(* Logix 5000 AddOnInstructionDefinition export Banner_IOL_Parameter_v6; software revision 33.00 *)

TYPE Banner_IOL_Device_Index_v6 :
STRUCT
   Index : Banner_IOL_Device_SubIndex_v6[41];
END_STRUCT
END_TYPE

TYPE Banner_IOL_Device_SubIndex_v6 :
STRUCT
   Sub : DINT[34];
END_STRUCT
END_TYPE

TYPE Banner_IOL_Device_v6 :
STRUCT
   Initial_Global_Read : BOOL;
   Command : SINT;
   Data : Banner_IOL_Device_Index_v6;
   Reset : BOOL;
END_STRUCT
END_TYPE

TYPE Banner_IOL_Port_v6 :   // UDT that has all of the data items necessary to communicate with a specific Port on a IO-Link Master
STRUCT
   Port_Controlled : INT;   // Each bit represents a port on an IO-Link Master. Set to 1 to tell AOI to control that port.
   Port_Activate : INT;   // Each bit represents a port on an IO-Link Master. When ON that port will process any commands in queue.
   Port_Read : INT;   // Each bit represents a port on an IO-Link Master. Used to determine when device AOI has requested a Read command.
   Port_Write : INT;   // Each bit represents a port on an IO-Link Master. Used to determine when device AOI has requested a Write command.
   Port_RW_Complete : INT;   // Each bit represents a port on an IO-Link Master. Tells device AOI that Read or Write request has been completed.
   Port_Device_Read : INT;
   Data_Transfer : SINT[250];   // Array to transfer data from IO-Master to device AOIs.
END_STRUCT
END_TYPE

TYPE Banner_IOL_Rules_Array_v6 :
STRUCT
   Length : DINT;
   Settings : Banner_IOL_Rules_SettingsArray_v6[41];
END_STRUCT
END_TYPE

TYPE Banner_IOL_Rules_SettingsArray_v6 :
STRUCT
   Index : DINT;
   Sub_Index : DINT;
   Num_Op : INT;   // Number of Operations to read/write Index.
   Total_Bytes : INT;
   RW : SINT;   // 0 = Read Only, 1 = Write Only, 2 = Read or Write
   Rules : Banner_IOL_Rules_v6[34];   // Sub Index Position in IODD.
END_STRUCT
END_TYPE

TYPE Banner_IOL_Rules_v6 :
STRUCT
   Byte_Pos : SINT;   // Byte Position to read from or write data to.
   Multi : SINT;   // Determines if a multiple byte length index is being accessed. Use 2 for 2 bytes length, 3 for 3 byte length, etc..
   BitControl : BOOL;   // 0=Standard byte control, 1=Bitwise packaging
   BitPos : SINT;   // Bit start position for operation
   BitValue : SINT;
   Sub_Index : SINT;
   Signed : SINT;   // 0=Unsigned, 1=Signed
END_STRUCT
END_TYPE

ADD_ON_INSTRUCTION Banner_IOL_Parameter_v6   (* revision 6.0 *)
// AOI that reads and writes to an IO-Link devices parameter data.
VAR_IN_OUT
   Device : Banner_IOL_Device_v6; {required}
   Rules : Banner_IOL_Rules_Array_v6; {required}
   Port_Data : Banner_IOL_Port_v6; {required}
END_VAR
VAR_INPUT
   Port : DINT; {required}
END_VAR
VAR_OUTPUT
   Done : BOOL; {access Read Only, visible}
   Busy : BOOL; {access Read Only, visible}
END_VAR
VAR
   Control : DINT; {access None}
   Inprocess_Index : INT; {access None}
   Index_Write_Inprocess : INT; {access None}
   Index_Write_Control : INT; {access None}
   Global_Read_Command : INT; {access None}
   Command_Being_Processed : BOOL; {access None}
   r_dex2 : INT; {access None}
   r_dex1 : INT; {access None}
   g_index : INT; {access None}
   r_dex3 : INT; {access None}
   r_dex4 : INT; {access None}
   r_dex5 : INT; {access None}
   Wr_Upper : INT; {access None}
   w_dex5 : INT; {access None}
   w_dex4 : INT; {access None}
   w_dex3 : INT; {access None}
   w_dex2 : INT; {access None}
   w_dex1 : INT; {access None}
   m3 : INT; {access None}
   m2 : INT; {access None}
   m1 : INT; {access None}
   b_dex : INT; {access None}
   GlobalCon : DINT; {access None}
   Signed : INT; {access None}
   Temp_Int : INT; {access None}
   Temp_Write : DINT; {access None}
   Temp_Read : DINT; {access None}
   Temp : DINT[10]; {access None}
END_VAR

ROUTINE Logic   (* ladder *)
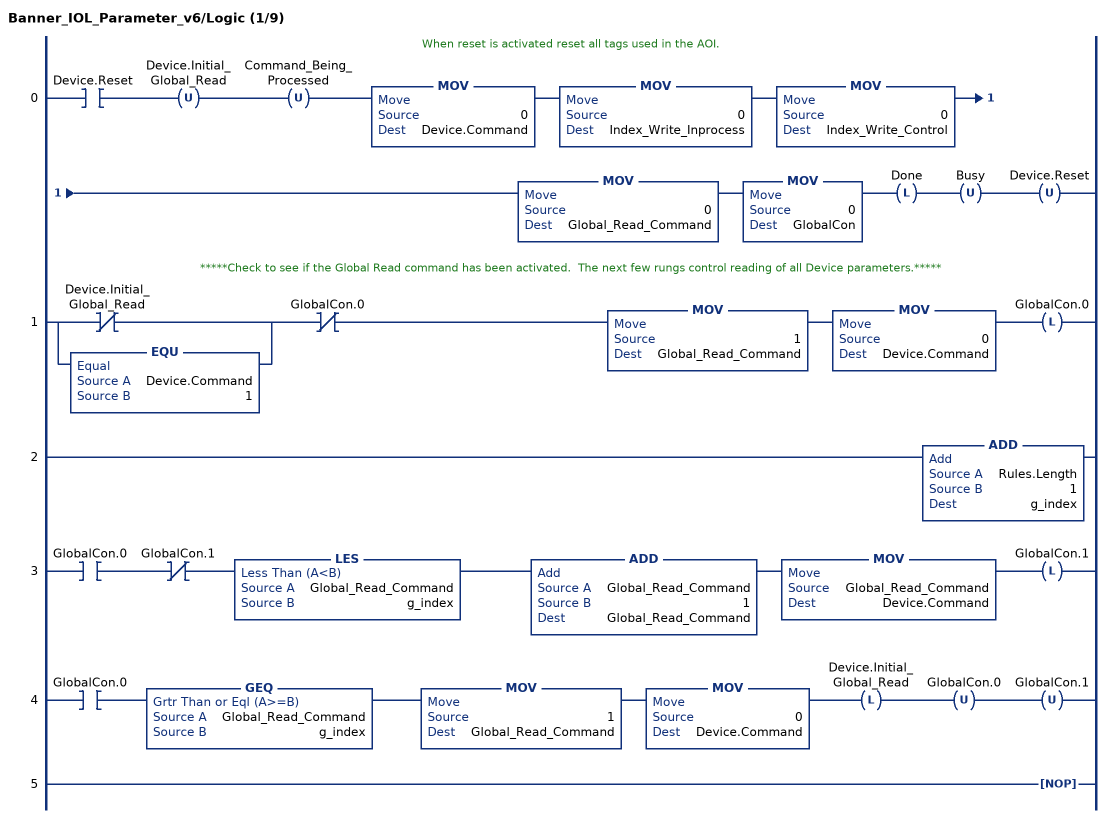
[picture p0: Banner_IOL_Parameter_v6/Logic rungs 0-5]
   // When reset is activated reset all tags used in the AOI.
   0: XIC(Device.Reset)OTU(Device.Initial_Global_Read)OTU(Command_Being_Processed)MOV(0,Device.Command)MOV(0,Index_Write_Inprocess)MOV(0,Index_Write_Control)MOV(0,Global_Read_Command)MOV(0,GlobalCon)OTL(Done)OTU(Busy)OTU(Device.Reset);
   // *****Check to see if the Global Read command has been activated.  The next few rungs control reading of all Device parameters.*****
   1: [XIO(Device.Initial_Global_Read) ,EQU(Device.Command,1) ]XIO(GlobalCon.0)MOV(1,Global_Read_Command)MOV(0,Device.Command)OTL(GlobalCon.0);
   2: ADD(Rules.Length,1,g_index);
   3: XIC(GlobalCon.0)XIO(GlobalCon.1)LES(Global_Read_Command,g_index)ADD(Global_Read_Command,1,Global_Read_Command)MOV(Global_Read_Command,Device.Command)OTL(GlobalCon.1);
   4: XIC(GlobalCon.0)GEQ(Global_Read_Command,g_index)MOV(1,Global_Read_Command)MOV(0,Device.Command)OTL(Device.Initial_Global_Read)OTU(GlobalCon.0)OTU(GlobalCon.1);
   5: NOP();
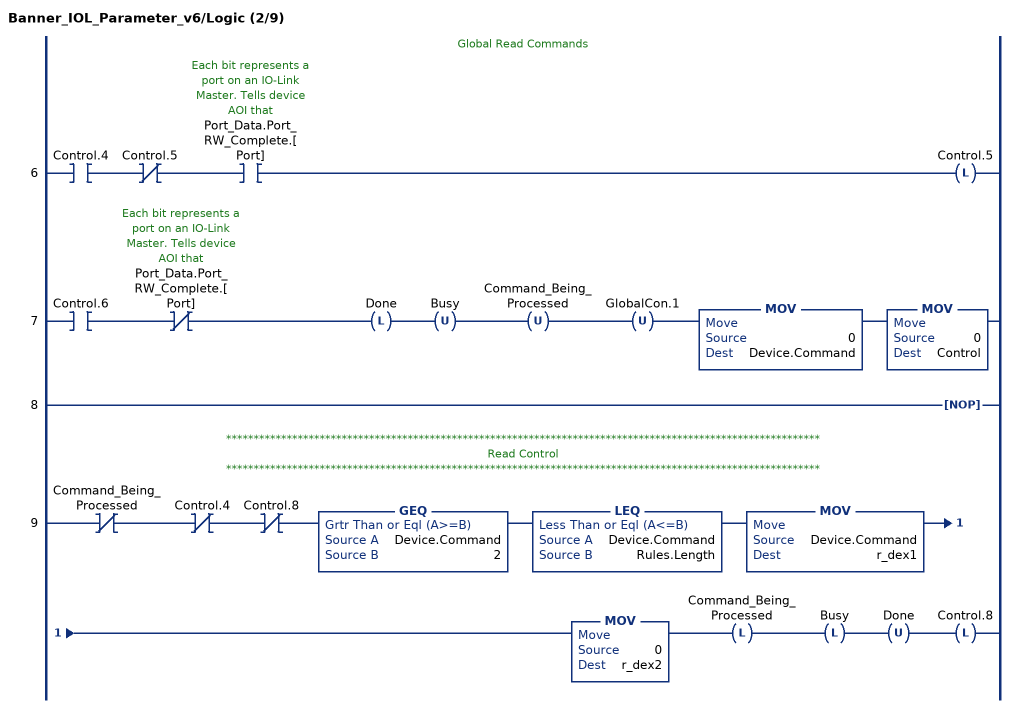
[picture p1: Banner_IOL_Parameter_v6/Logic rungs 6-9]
   // Global Read Commands
   6: XIC(Control.4)XIO(Control.5)XIC(Port_Data.Port_RW_Complete.[Port])OTL(Control.5);
   7: XIC(Control.6)XIO(Port_Data.Port_RW_Complete.[Port])OTL(Done)OTU(Busy)OTU(Command_Being_Processed)OTU(GlobalCon.1)MOV(0,Device.Command)MOV(0,Control);
   8: NOP();
   // ************************************************************************************************************
   // Read Control
   // ************************************************************************************************************
   9: XIO(Command_Being_Processed)XIO(Control.4)XIO(Control.8)GEQ(Device.Command,2)LEQ(Device.Command,Rules.Length)MOV(Device.Command,r_dex1)MOV(0,r_dex2)OTL(Command_Being_Processed)OTL(Busy)OTU(Done)OTL(Control.8);
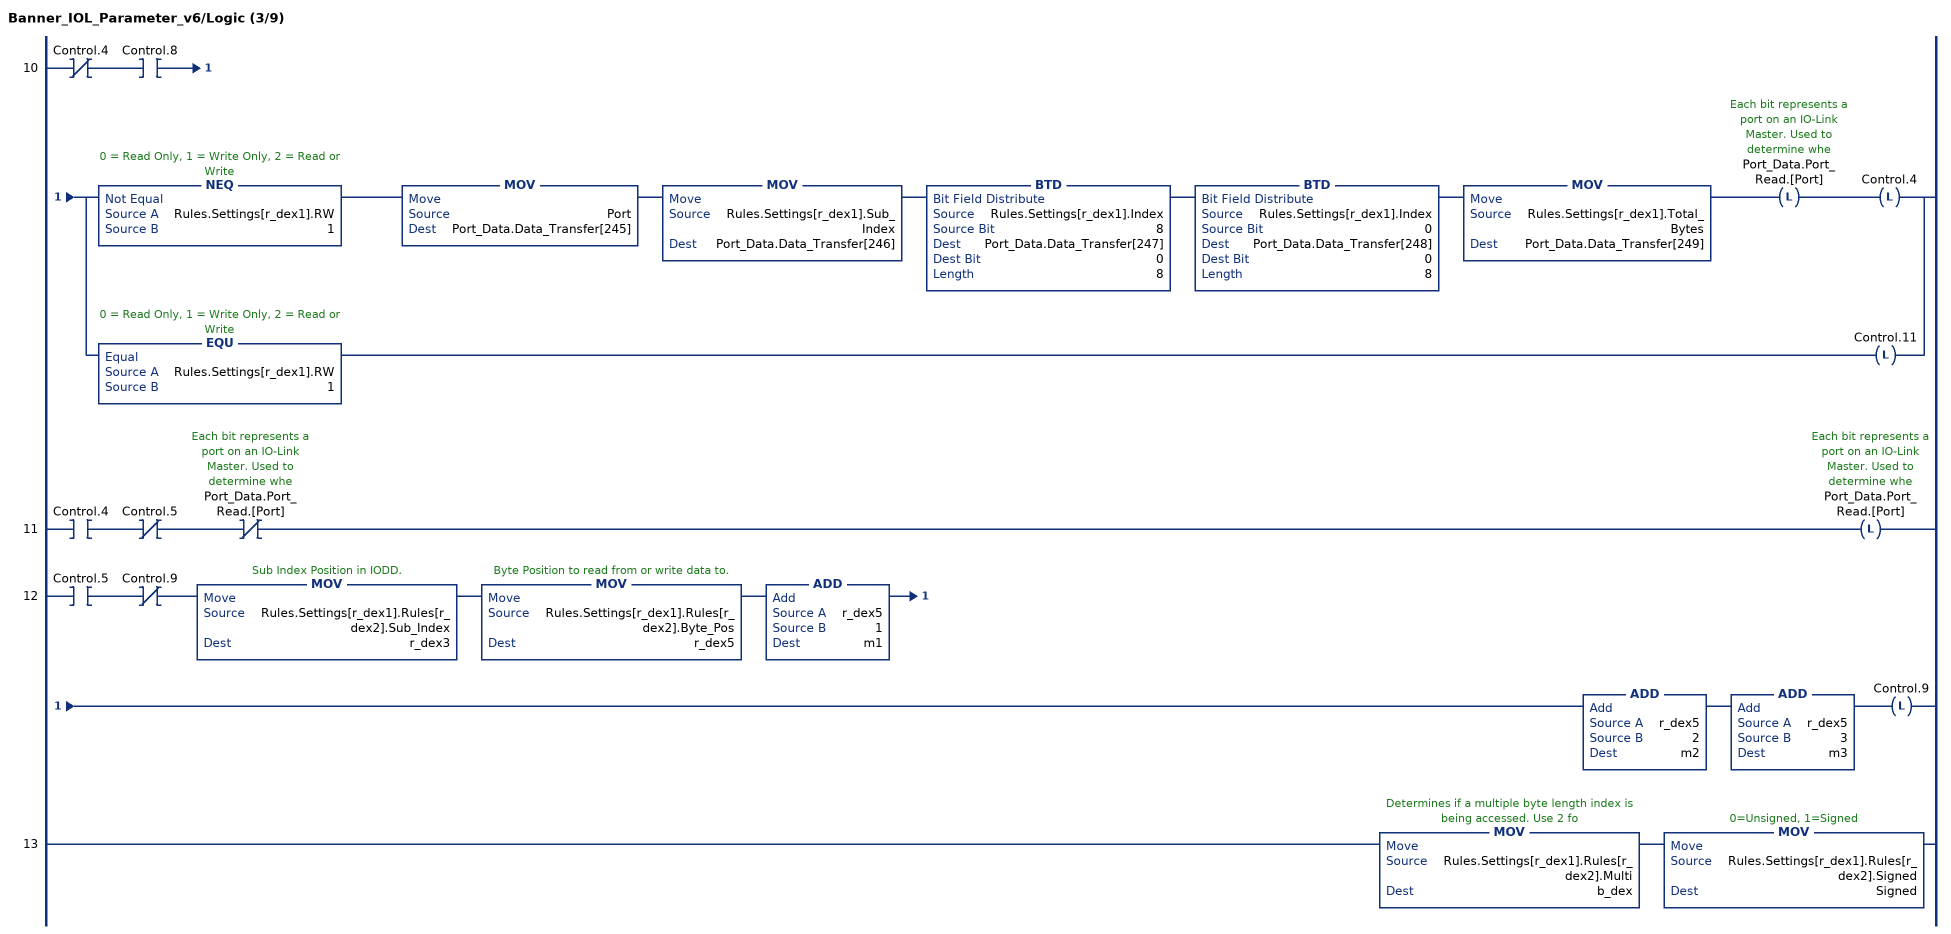
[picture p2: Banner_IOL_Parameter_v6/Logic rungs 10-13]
   10: XIO(Control.4)XIC(Control.8)[NEQ(Rules.Settings[r_dex1].RW,1) MOV(Port,Port_Data.Data_Transfer[245]) MOV(Rules.Settings[r_dex1].Sub_Index,Port_Data.Data_Transfer[246]) BTD(Rules.Settings[r_dex1].Index,8,Port_Data.Data_Transfer[247],0,8) BTD(Rules.Settings[r_dex1].Index,0,Port_Data.Data_Transfer[248],0,8) MOV(Rules.Settings[r_dex1].Total_Bytes,Port_Data.Data_Transfer[249]) OTL(Port_Data.Port_Read.[Port]) OTL(Control.4) ,EQU(Rules.Settings[r_dex1].RW,1) OTL(Control.11) ];
   11: XIC(Control.4)XIO(Control.5)XIO(Port_Data.Port_Read.[Port])OTL(Port_Data.Port_Read.[Port]);
   12: XIC(Control.5)XIO(Control.9)MOV(Rules.Settings[r_dex1].Rules[r_dex2].Sub_Index,r_dex3)MOV(Rules.Settings[r_dex1].Rules[r_dex2].Byte_Pos,r_dex5)ADD(r_dex5,1,m1)ADD(r_dex5,2,m2)ADD(r_dex5,3,m3)OTL(Control.9);
   13: MOV(Rules.Settings[r_dex1].Rules[r_dex2].Multi,b_dex)MOV(Rules.Settings[r_dex1].Rules[r_dex2].Signed,Signed);
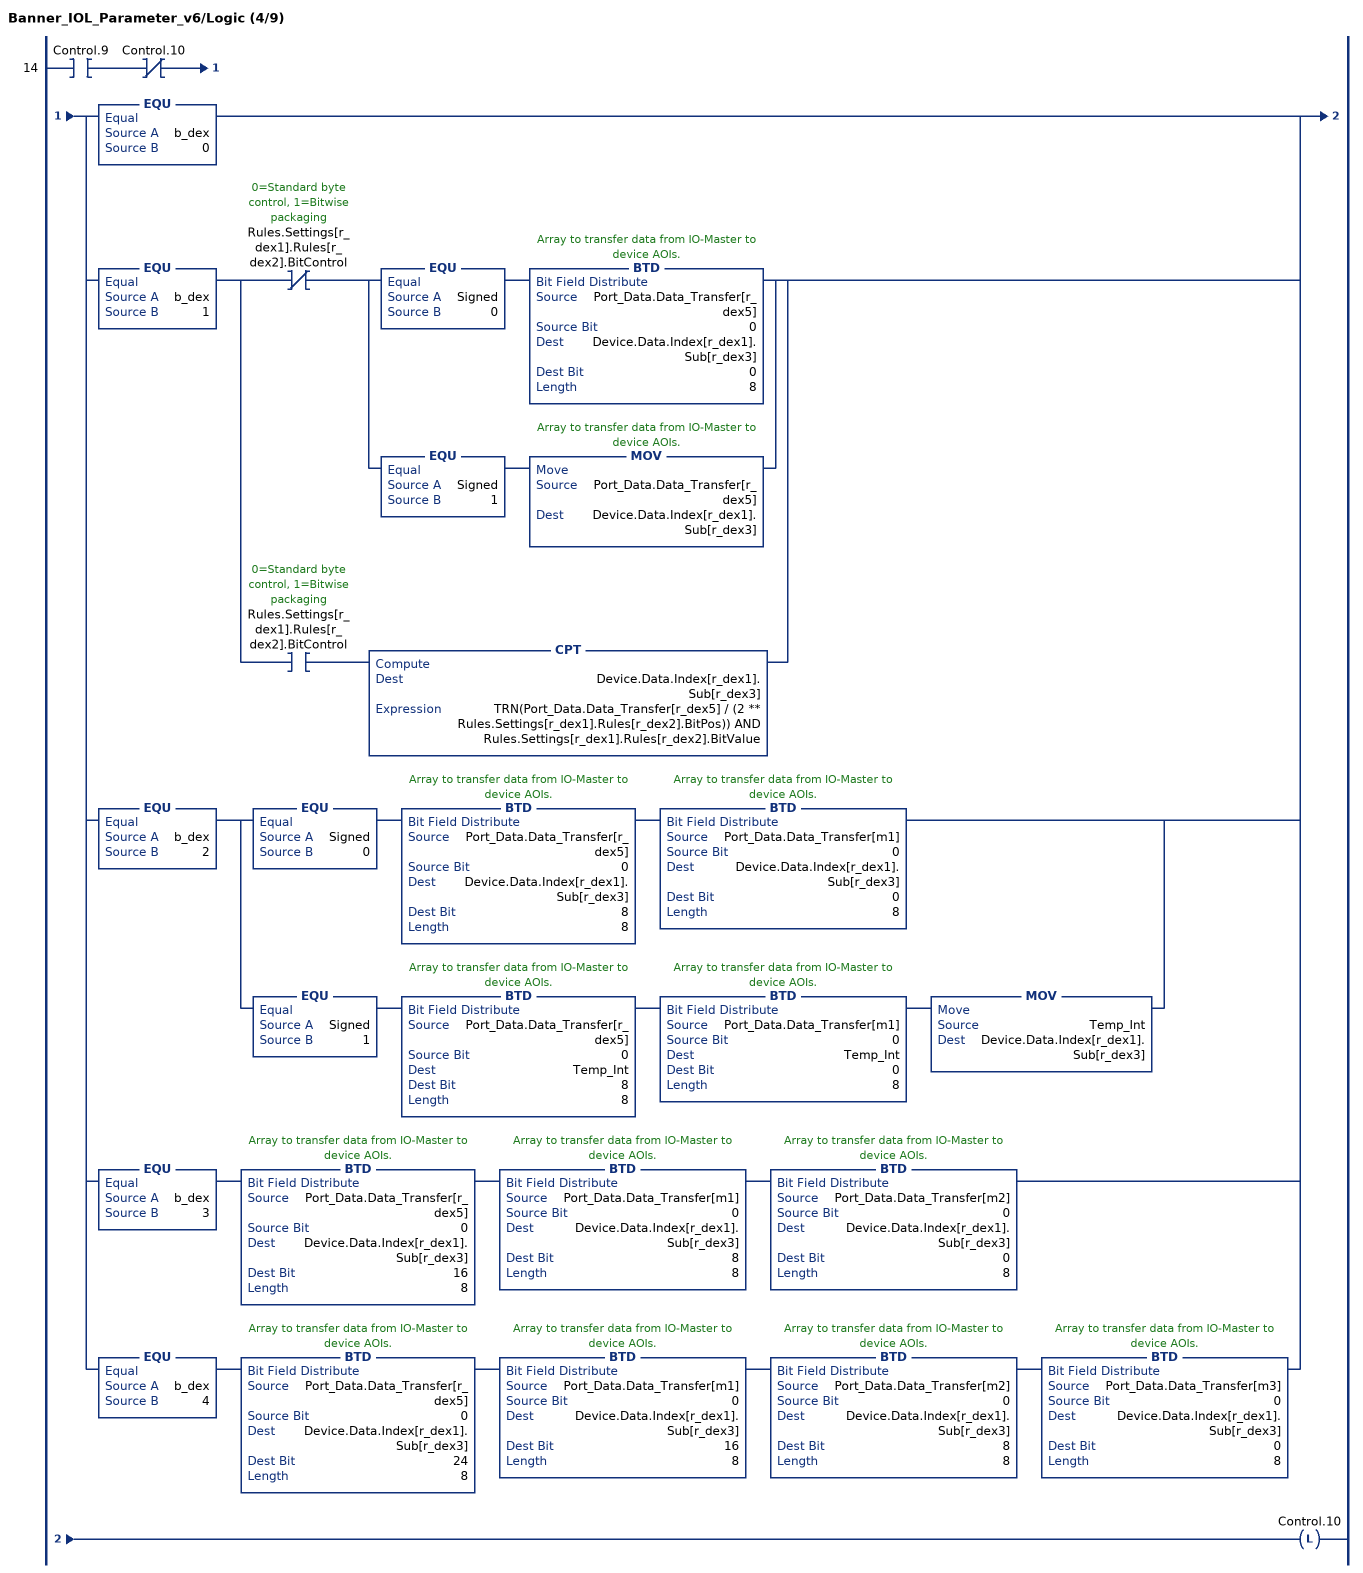
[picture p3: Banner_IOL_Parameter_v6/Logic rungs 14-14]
   14: XIC(Control.9)XIO(Control.10)[EQU(b_dex,0) ,EQU(b_dex,1) [XIO(Rules.Settings[r_dex1].Rules[r_dex2].BitControl) [EQU(Signed,0) BTD(Port_Data.Data_Transfer[r_dex5],0,Device.Data.Index[r_dex1].Sub[r_dex3],0,8) ,EQU(Signed,1) MOV(Port_Data.Data_Transfer[r_dex5],Device.Data.Index[r_dex1].Sub[r_dex3]) ] ,XIC(Rules.Settings[r_dex1].Rules[r_dex2].BitControl) CPT(Device.Data.Index[r_dex1].Sub[r_dex3],TRN(Port_Data.Data_Transfer[r_dex5] / (2 ** Rules.Settings[r_dex1].Rules[r_dex2].BitPos)) AND Rules.Settings[r_dex1].Rules[r_dex2].BitValue) ] ,EQU(b_dex,2) [EQU(Signed,0) BTD(Port_Data.Data_Transfer[r_dex5],0,Device.Data.Index[r_dex1].Sub[r_dex3],8,8) BTD(Port_Data.Data_Transfer[m1],0,Device.Data.Index[r_dex1].Sub[r_dex3],0,8) ,EQU(Signed,1) BTD(Port_Data.Data_Transfer[r_dex5],0,Temp_Int,8,8) BTD(Port_Data.Data_Transfer[m1],0,Temp_Int,0,8) MOV(Temp_Int,Device.Data.Index[r_dex1].Sub[r_dex3]) ] ,EQU(b_dex,3) BTD(Port_Data.Data_Transfer[r_dex5],0,Device.Data.Index[r_dex1].Sub[r_dex3],16,8) BTD(Port_Data.Data_Transfer[m1],0,Device.Data.Index[r_dex1].Sub[r_dex3],8,8) BTD(Port_Data.Data_Transfer[m2],0,Device.Data.Index[r_dex1].Sub[r_dex3],0,8) ,EQU(b_dex,4) BTD(Port_Data.Data_Transfer[r_dex5],0,Device.Data.Index[r_dex1].Sub[r_dex3],24,8) BTD(Port_Data.Data_Transfer[m1],0,Device.Data.Index[r_dex1].Sub[r_dex3],16,8) BTD(Port_Data.Data_Transfer[m2],0,Device.Data.Index[r_dex1].Sub[r_dex3],8,8) BTD(Port_Data.Data_Transfer[m3],0,Device.Data.Index[r_dex1].Sub[r_dex3],0,8) ]OTL(Control.10);
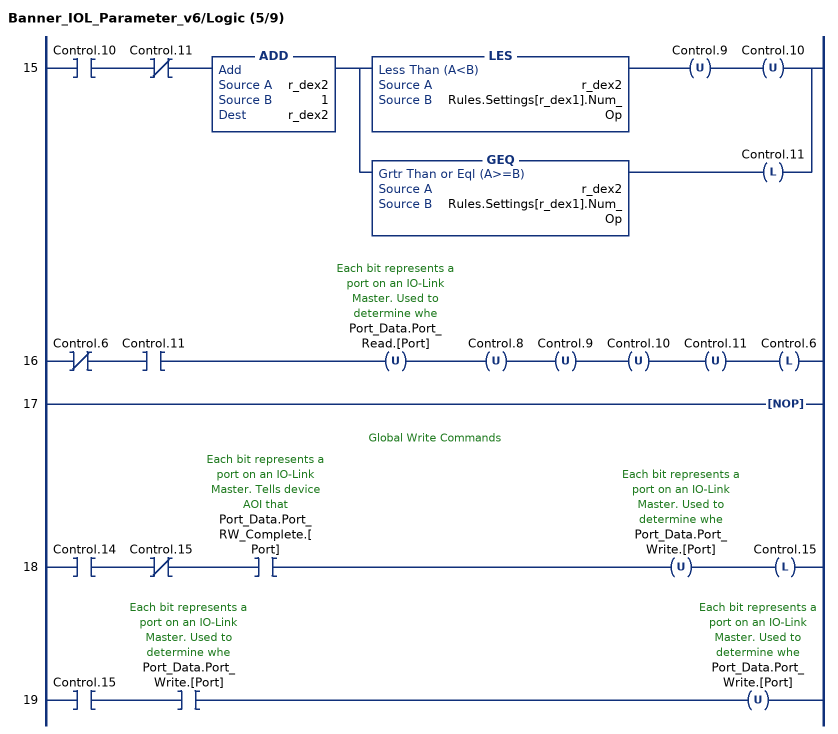
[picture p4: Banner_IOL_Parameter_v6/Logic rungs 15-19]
   15: XIC(Control.10)XIO(Control.11)ADD(r_dex2,1,r_dex2)[LES(r_dex2,Rules.Settings[r_dex1].Num_Op) OTU(Control.9) OTU(Control.10) ,GEQ(r_dex2,Rules.Settings[r_dex1].Num_Op) OTL(Control.11) ];
   16: XIO(Control.6)XIC(Control.11)OTU(Port_Data.Port_Read.[Port])OTU(Control.8)OTU(Control.9)OTU(Control.10)OTU(Control.11)OTL(Control.6);
   17: NOP();
   // Global Write Commands
   18: XIC(Control.14)XIO(Control.15)XIC(Port_Data.Port_RW_Complete.[Port])OTU(Port_Data.Port_Write.[Port])OTL(Control.15);
   19: XIC(Control.15)XIC(Port_Data.Port_Write.[Port])OTU(Port_Data.Port_Write.[Port]);
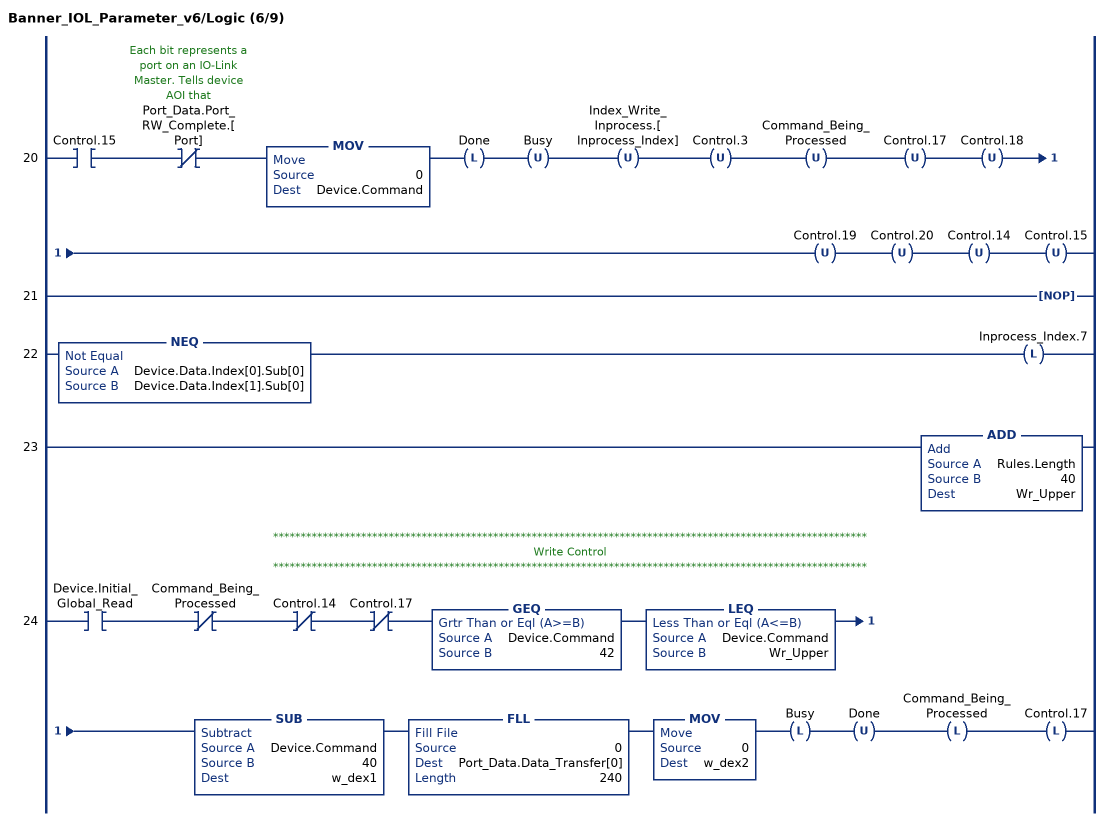
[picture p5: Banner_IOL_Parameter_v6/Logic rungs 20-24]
   20: XIC(Control.15)XIO(Port_Data.Port_RW_Complete.[Port])MOV(0,Device.Command)OTL(Done)OTU(Busy)OTU(Index_Write_Inprocess.[Inprocess_Index])OTU(Control.3)OTU(Command_Being_Processed)OTU(Control.17)OTU(Control.18)OTU(Control.19)OTU(Control.20)OTU(Control.14)OTU(Control.15);
   21: NOP();
   22: NEQ(Device.Data.Index[0].Sub[0],Device.Data.Index[1].Sub[0])OTL(Inprocess_Index.7);
   23: ADD(Rules.Length,40,Wr_Upper);
   // ************************************************************************************************************
   // Write Control
   // ************************************************************************************************************
   24: XIC(Device.Initial_Global_Read)XIO(Command_Being_Processed)XIO(Control.14)XIO(Control.17)GEQ(Device.Command,42)LEQ(Device.Command,Wr_Upper)SUB(Device.Command,40,w_dex1)FLL(0,Port_Data.Data_Transfer[0],240)MOV(0,w_dex2)OTL(Busy)OTU(Done)OTL(Command_Being_Processed)OTL(Control.17);
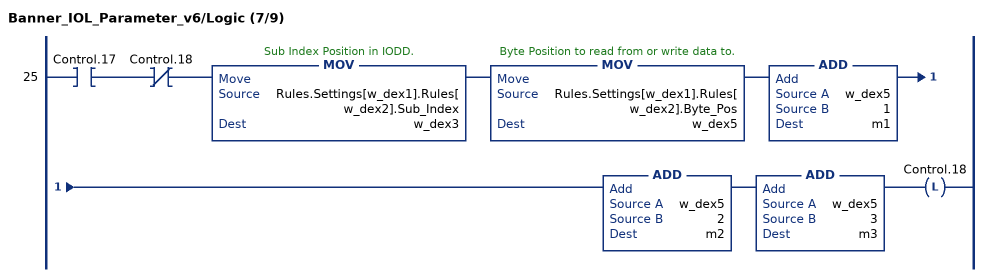
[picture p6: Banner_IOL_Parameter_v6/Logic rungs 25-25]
   25: XIC(Control.17)XIO(Control.18)MOV(Rules.Settings[w_dex1].Rules[w_dex2].Sub_Index,w_dex3)MOV(Rules.Settings[w_dex1].Rules[w_dex2].Byte_Pos,w_dex5)ADD(w_dex5,1,m1)ADD(w_dex5,2,m2)ADD(w_dex5,3,m3)OTL(Control.18);
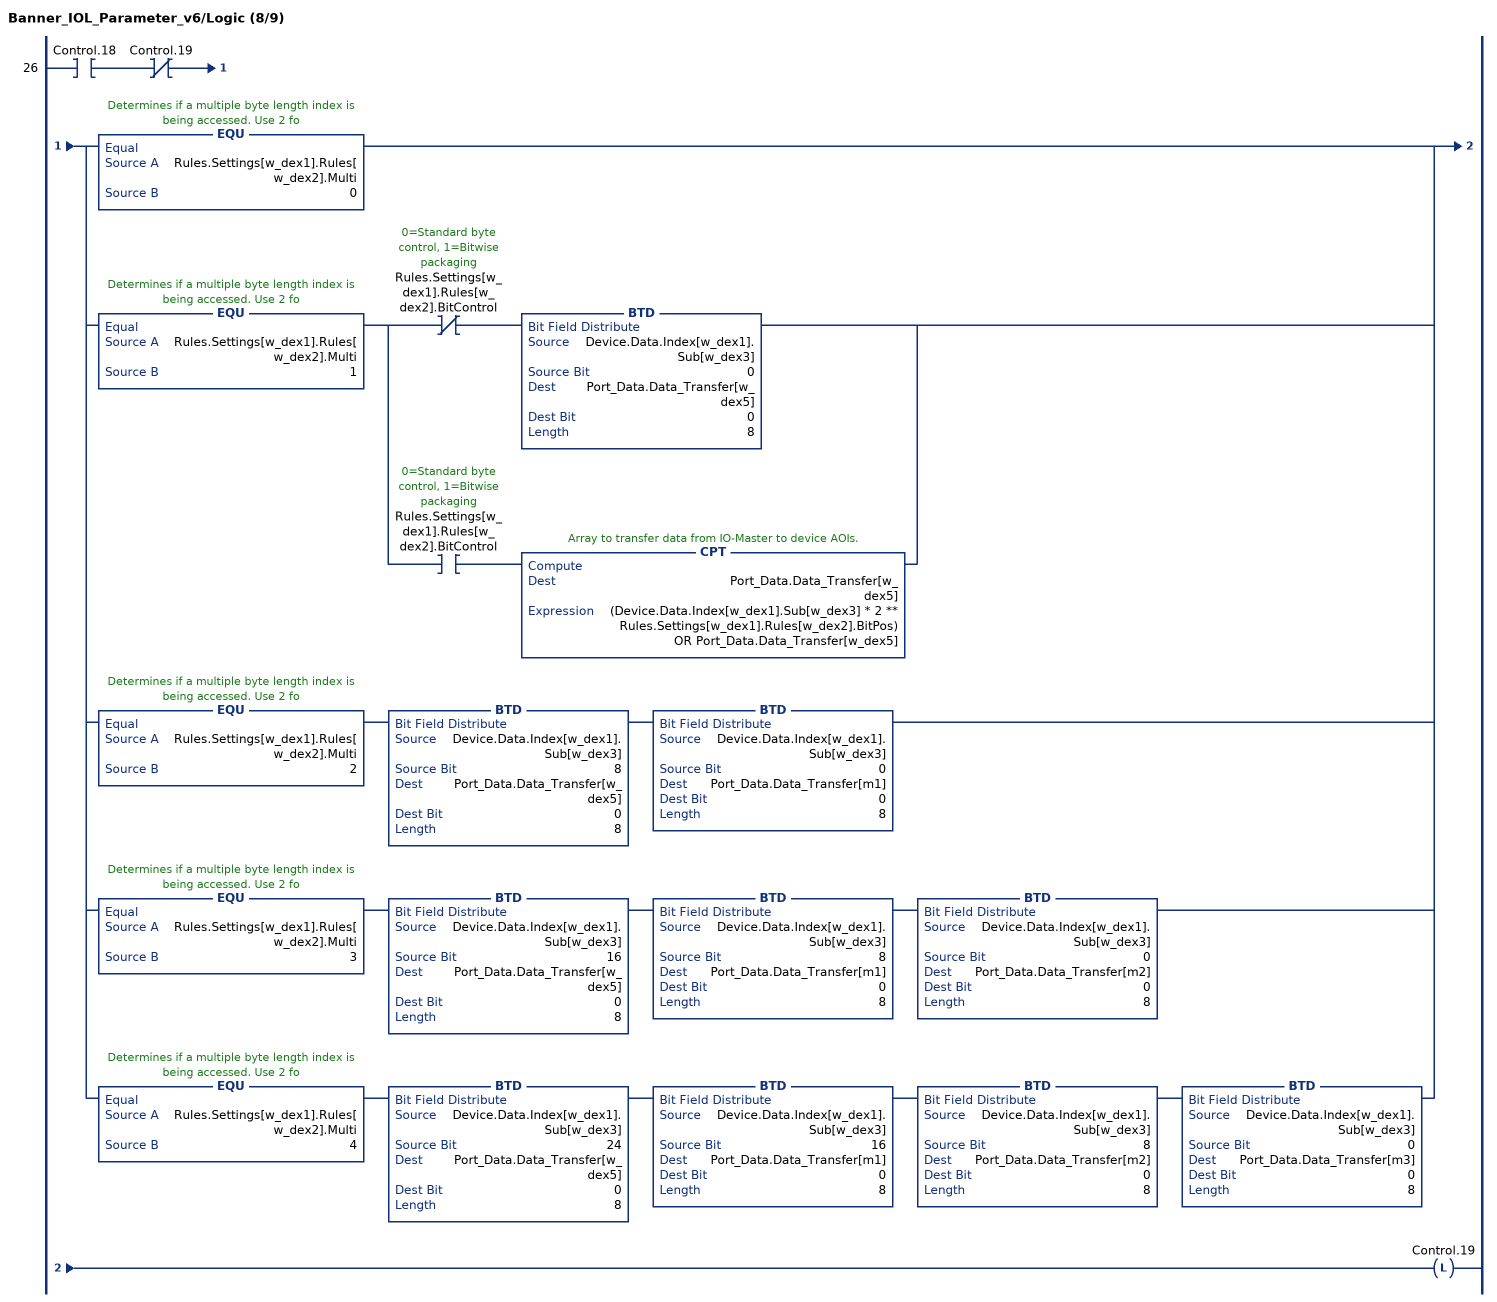
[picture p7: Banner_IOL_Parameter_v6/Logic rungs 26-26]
   26: XIC(Control.18)XIO(Control.19)[EQU(Rules.Settings[w_dex1].Rules[w_dex2].Multi,0) ,EQU(Rules.Settings[w_dex1].Rules[w_dex2].Multi,1) [XIO(Rules.Settings[w_dex1].Rules[w_dex2].BitControl) BTD(Device.Data.Index[w_dex1].Sub[w_dex3],0,Port_Data.Data_Transfer[w_dex5],0,8) ,XIC(Rules.Settings[w_dex1].Rules[w_dex2].BitControl) CPT(Port_Data.Data_Transfer[w_dex5],(Device.Data.Index[w_dex1].Sub[w_dex3] * 2 ** Rules.Settings[w_dex1].Rules[w_dex2].BitPos) OR Port_Data.Data_Transfer[w_dex5]) ] ,EQU(Rules.Settings[w_dex1].Rules[w_dex2].Multi,2) BTD(Device.Data.Index[w_dex1].Sub[w_dex3],8,Port_Data.Data_Transfer[w_dex5],0,8) BTD(Device.Data.Index[w_dex1].Sub[w_dex3],0,Port_Data.Data_Transfer[m1],0,8) ,EQU(Rules.Settings[w_dex1].Rules[w_dex2].Multi,3) BTD(Device.Data.Index[w_dex1].Sub[w_dex3],16,Port_Data.Data_Transfer[w_dex5],0,8) BTD(Device.Data.Index[w_dex1].Sub[w_dex3],8,Port_Data.Data_Transfer[m1],0,8) BTD(Device.Data.Index[w_dex1].Sub[w_dex3],0,Port_Data.Data_Transfer[m2],0,8) ,EQU(Rules.Settings[w_dex1].Rules[w_dex2].Multi,4) BTD(Device.Data.Index[w_dex1].Sub[w_dex3],24,Port_Data.Data_Transfer[w_dex5],0,8) BTD(Device.Data.Index[w_dex1].Sub[w_dex3],16,Port_Data.Data_Transfer[m1],0,8) BTD(Device.Data.Index[w_dex1].Sub[w_dex3],8,Port_Data.Data_Transfer[m2],0,8) BTD(Device.Data.Index[w_dex1].Sub[w_dex3],0,Port_Data.Data_Transfer[m3],0,8) ]OTL(Control.19);
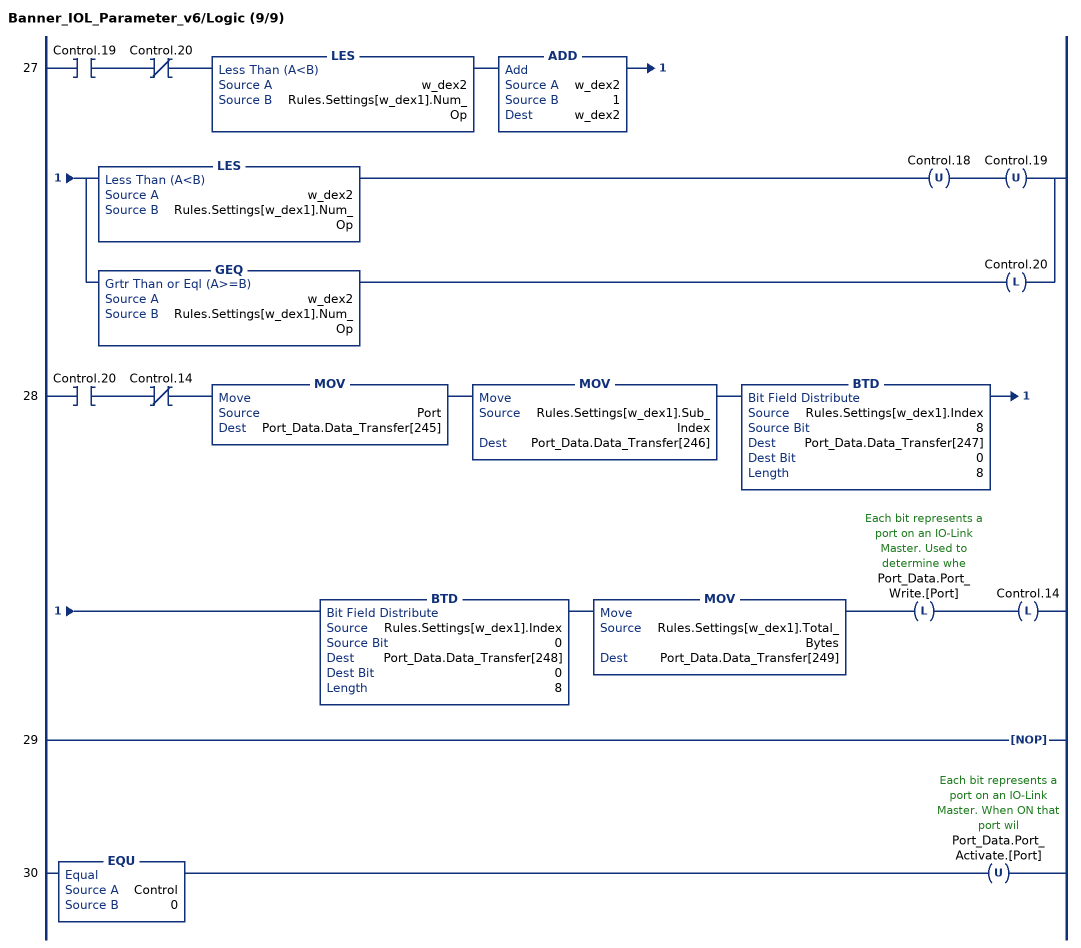
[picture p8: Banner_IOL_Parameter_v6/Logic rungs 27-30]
   27: XIC(Control.19)XIO(Control.20)LES(w_dex2,Rules.Settings[w_dex1].Num_Op)ADD(w_dex2,1,w_dex2)[LES(w_dex2,Rules.Settings[w_dex1].Num_Op) OTU(Control.18) OTU(Control.19) ,GEQ(w_dex2,Rules.Settings[w_dex1].Num_Op) OTL(Control.20) ];
   28: XIC(Control.20)XIO(Control.14)MOV(Port,Port_Data.Data_Transfer[245])MOV(Rules.Settings[w_dex1].Sub_Index,Port_Data.Data_Transfer[246])BTD(Rules.Settings[w_dex1].Index,8,Port_Data.Data_Transfer[247],0,8)BTD(Rules.Settings[w_dex1].Index,0,Port_Data.Data_Transfer[248],0,8)MOV(Rules.Settings[w_dex1].Total_Bytes,Port_Data.Data_Transfer[249])OTL(Port_Data.Port_Write.[Port])OTL(Control.14);
   29: NOP();
   30: EQU(Control,0)OTU(Port_Data.Port_Activate.[Port]);
END_ROUTINE
END_ADD_ON_INSTRUCTION
